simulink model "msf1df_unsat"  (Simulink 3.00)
settings: Solver=ode45  SolverMode=SingleTasking  StartTime=0.0  StopTime=30  MaxStep=10  RelTol=1e-5  AbsTol=1e-6
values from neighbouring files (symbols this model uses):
  Disturb = Setpoint    [mimo_MSF1DF_sim.m]    (also in mimo_MSF2DF_sim.m)
  K = 1/kpd    [imc2pseucon.m]    (also in imc2pseudo.m)
  Setpoint = zeros(1,n)    [mimo_MSF1DF_sim.m]    (also in mimo_MSF2DF_sim.m)
undefined symbols (not defined in the file or in its folder): denFs, denMs, denPd, denPs, Ksp, Md, Mdelay, Mnt, numFs, numPd, numPs, Pdelay
libraries: simulink3 x3

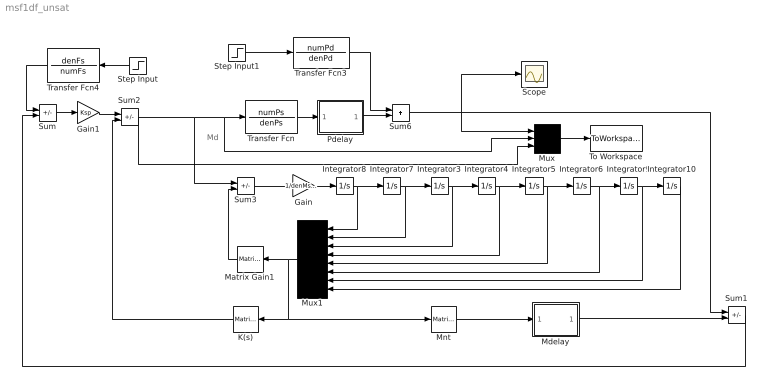
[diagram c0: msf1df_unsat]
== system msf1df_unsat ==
  note: Md
  Gain : Gain  Gain=1/denMs(1)  SaturateOnIntegerOverflow=on
  Gain1 : Gain  Gain=Ksp  SaturateOnIntegerOverflow=on
  Integrator{3..10} (8 alike) : Integrator  ExternalReset=none  InitialConditionSource=internal  InitialCondition=0  LimitOutput=off  UpperSaturationLimit=inf  LowerSaturationLimit=-inf  ShowSaturationPort=off  ShowStatePort=off  AbsoluteTolerance=auto
  K(s) : simulink3/Math/Matrix Gain  Orientation=left  K=K(2:9)
  Matrix Gain1 : simulink3/Math/Matrix Gain  Orientation=left  K=Md(2:9)
  Mdelay : Subsystem
  Mnt : simulink3/Math/Matrix Gain  K=Mnt
  Mux : Mux  Inputs=3
  Mux1 : Mux  Orientation=left  Inputs=8
  Pdelay : Subsystem
  Scope : Scope
  Step Input : Step  Orientation=left  Time=0  Before=0  After=Setpoint  SampleTime=0
  Step Input1 : Step  Time=0  Before=0  After=Disturb  SampleTime=0
  Sum{,1..3} (4 alike) : Sum  Inputs=+-  SaturateOnIntegerOverflow=on
  Sum6 : Sum  Inputs=++  SaturateOnIntegerOverflow=on
  To Workspace : ToWorkspace  VariableName=simout  SampleTime=-1  SaveFormat=Matrix
  Transfer Fcn : TransferFcn  Numerator=numPs  Denominator=denPs
  Transfer Fcn3 : TransferFcn  Numerator=numPd  Denominator=denPd
  Transfer Fcn4 : TransferFcn  Orientation=left  Numerator=denFs  Denominator=numFs
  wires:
  Step Input1/1 -> Transfer Fcn3/1
  Transfer Fcn3/1 -> Sum6/1
  Pdelay/1(Out1) -> Sum6/2
  Mux/1 -> To Workspace/1
  Transfer Fcn/1 -> Pdelay/1(In1)
  Gain1/1 -> Sum2/1
  Sum/1 -> Gain1/1
  Sum6/1 -> Mux/1, Sum1/1, Scope/1
  Gain/1 -> Integrator8/1
  Sum3/1 -> Gain/1
  Matrix Gain1/1 -> Sum3/2
  Mnt/1 -> Mdelay/1(In1)
  Mdelay/1(Out1) -> Sum1/2
  Sum1/1 -> Sum/2
  K(s)/1 -> Sum2/2
  Step Input/1 -> Transfer Fcn4/1
  Transfer Fcn4/1 -> Sum/1
  Integrator8/1 -> Integrator7/1, Mux1/1
  Mux1/1 -> Matrix Gain1/1, Mnt/1, K(s)/1
  Integrator7/1 -> Integrator3/1, Mux1/2
  Integrator3/1 -> Integrator4/1, Mux1/3
  Integrator4/1 -> Integrator5/1, Mux1/4
  Integrator5/1 -> Integrator6/1, Mux1/5
  Integrator6/1 -> Integrator9/1, Mux1/6
  Integrator9/1 -> Integrator10/1, Mux1/7
  Integrator10/1 -> Mux1/8
  Sum2/1 -> Mux/3, Sum3/1, Transfer Fcn/1, Mux/2

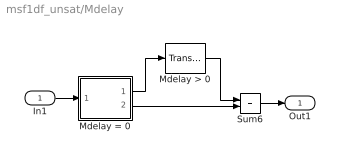
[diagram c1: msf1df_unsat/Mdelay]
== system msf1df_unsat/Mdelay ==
  In1 : Inport  Port=1  PortWidth=-1  SampleTime=-1  DataType=auto
  Mdelay > 0 : TransportDelay  DelayTime=Mdelay  InitialInput=0  BufferSize=1024
  Mdelay = 0 : Subsystem  Description=pass input signal through out1 if condition is true.
  Sum6 : Sum  Inputs=++  SaturateOnIntegerOverflow=on
  Out1 : Outport  Port=1
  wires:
  Mdelay = 0/1(Out2) -> Mdelay > 0/1
  Mdelay > 0/1 -> Sum6/1
  Mdelay = 0/2(Out1) -> Sum6/2
  In1/1 -> Mdelay = 0/1(In)
  Sum6/1 -> Out1/1

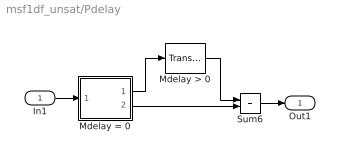
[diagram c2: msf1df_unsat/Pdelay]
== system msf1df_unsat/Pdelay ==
  In1 : Inport  Port=1  PortWidth=-1  SampleTime=-1  DataType=auto
  Mdelay > 0 : TransportDelay  DelayTime=Pdelay  InitialInput=0  BufferSize=1024
  Mdelay = 0 : Subsystem  Description=pass input signal through out1 if condition is true.
  Sum6 : Sum  Inputs=++  SaturateOnIntegerOverflow=on
  Out1 : Outport  Port=1
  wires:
  Mdelay = 0/1(Out2) -> Mdelay > 0/1
  Mdelay > 0/1 -> Sum6/1
  Mdelay = 0/2(Out1) -> Sum6/2
  In1/1 -> Mdelay = 0/1(In)
  Sum6/1 -> Out1/1

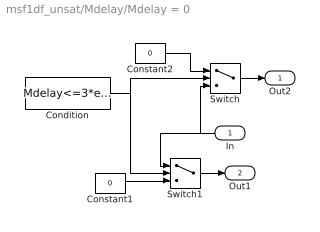
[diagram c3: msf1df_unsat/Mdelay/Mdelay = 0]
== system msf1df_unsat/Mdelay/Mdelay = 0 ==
  In : Inport  Orientation=left  Port=1  PortWidth=-1  SampleTime=-1  DataType=auto
  Condition : Constant  Value=Mdelay<=3*eps
  Constant1 : Constant  Value=0
  Constant2 : Constant  Value=0
  Switch : Switch  Threshold=1
  Switch1 : Switch  Threshold=1
  Out2 : Outport  Port=1  InitialOutput=0
  Out1 : Outport  Port=2  InitialOutput=0
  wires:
  In/1 -> Switch/3, Switch1/1
  Condition/1 -> Switch1/2, Switch/2
  Constant1/1 -> Switch1/3
  Constant2/1 -> Switch/1
  Switch/1 -> Out2/1
  Switch1/1 -> Out1/1

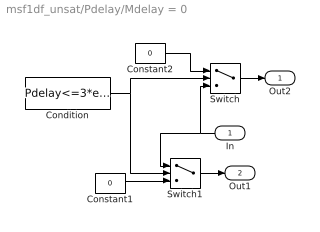
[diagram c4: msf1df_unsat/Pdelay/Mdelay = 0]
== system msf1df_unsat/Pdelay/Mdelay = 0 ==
  In : Inport  Orientation=left  Port=1  PortWidth=-1  SampleTime=-1  DataType=auto
  Condition : Constant  Value=Pdelay<=3*eps
  Constant1 : Constant  Value=0
  Constant2 : Constant  Value=0
  Switch : Switch  Threshold=1
  Switch1 : Switch  Threshold=1
  Out2 : Outport  Port=1  InitialOutput=0
  Out1 : Outport  Port=2  InitialOutput=0
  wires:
  In/1 -> Switch/3, Switch1/1
  Condition/1 -> Switch1/2, Switch/2
  Constant1/1 -> Switch1/3
  Constant2/1 -> Switch/1
  Switch/1 -> Out2/1
  Switch1/1 -> Out1/1
